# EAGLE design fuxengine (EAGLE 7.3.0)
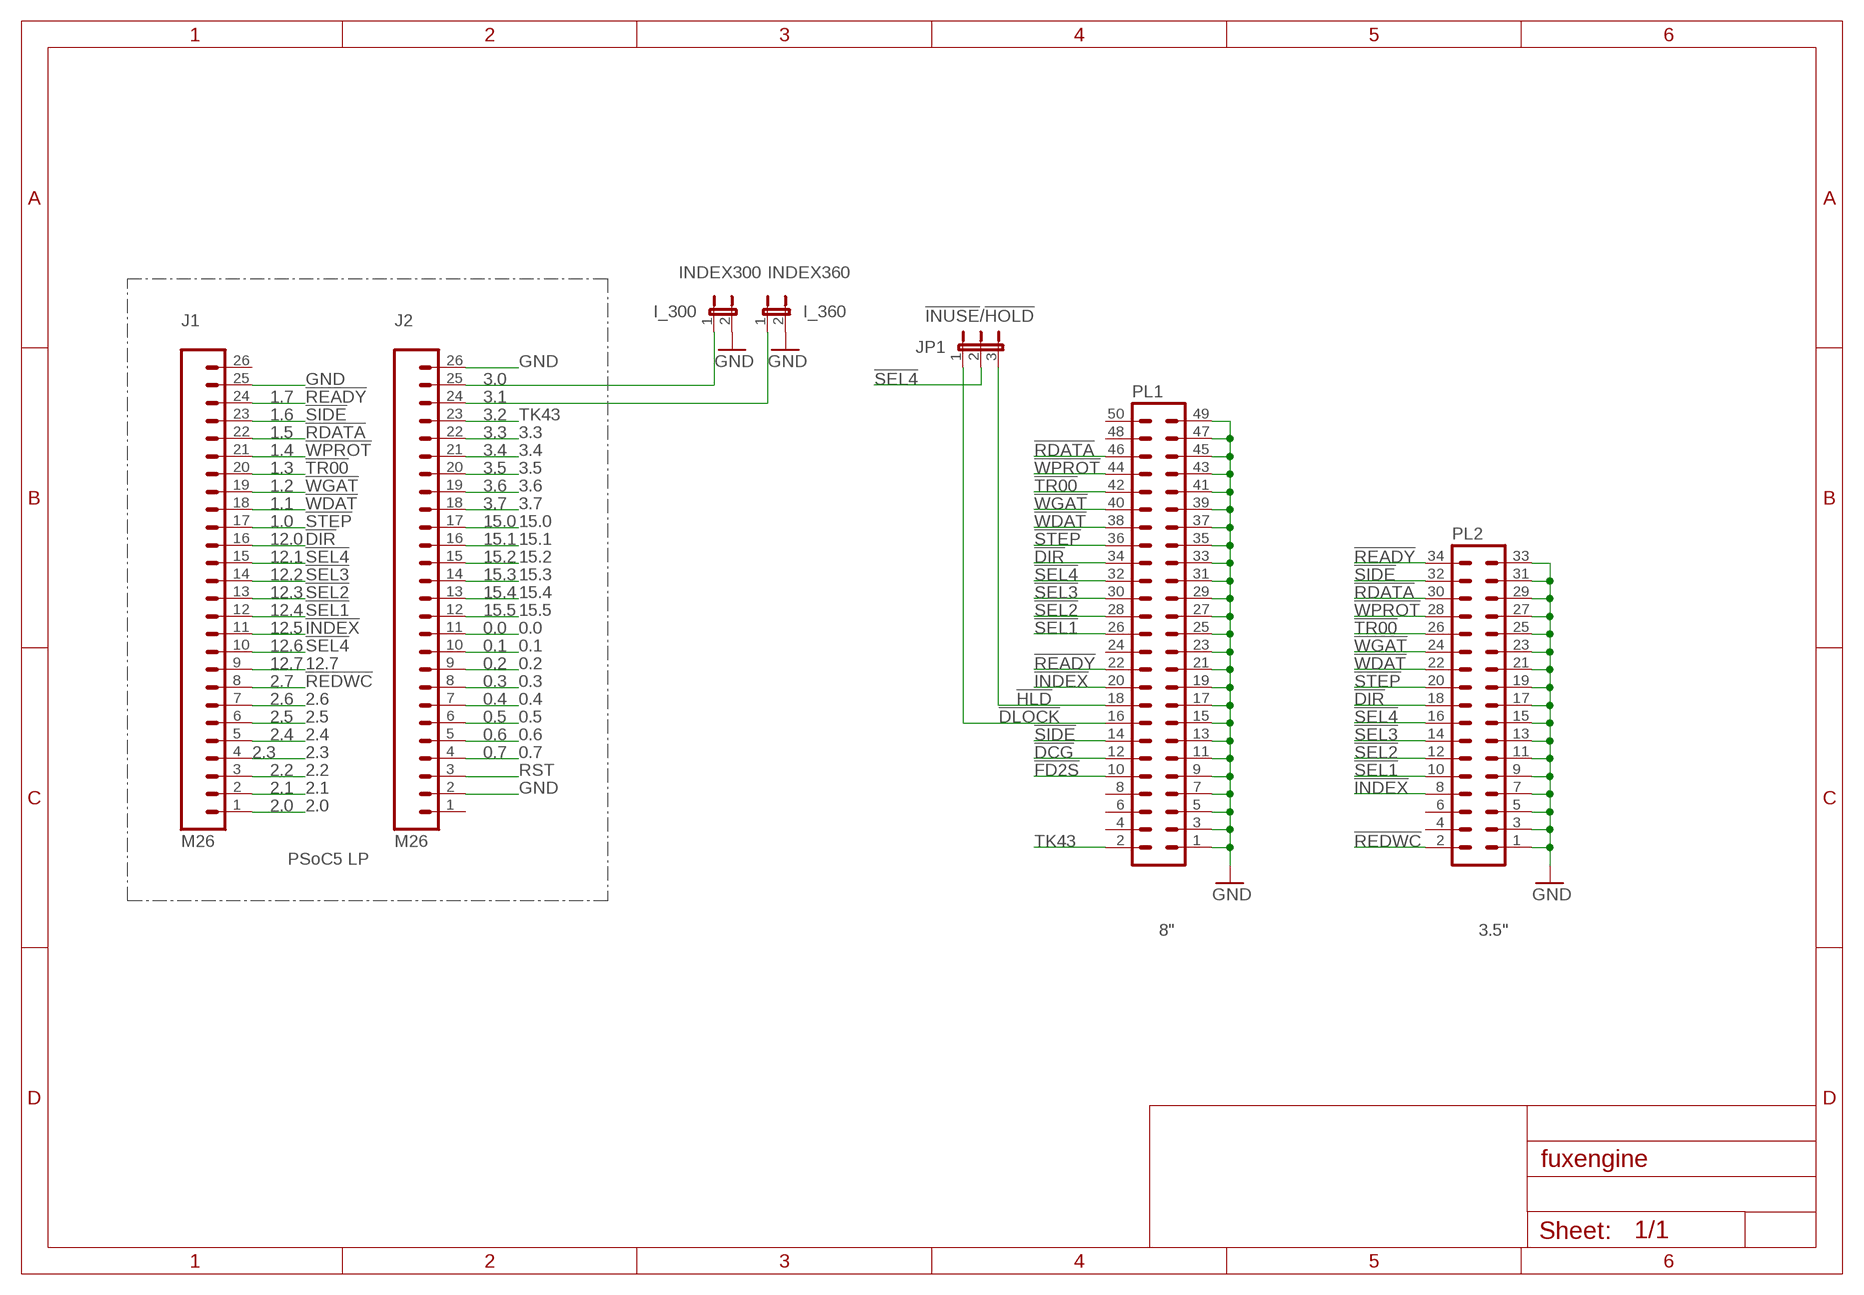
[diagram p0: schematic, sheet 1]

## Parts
I_300  JP1E  [JP1]
I_360  JP1E  [JP1]
J1  M26  [1X26]
J2  M26  [1X26]
JP1  !INUSE!/!HOLD  JP2E  [JP2]
PL1  50V  [50V]
PL2  34V  [34V]

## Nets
0.0: J2.11
0.1: J2.10
0.2: J2.9
0.3: J2.8
0.4: J2.7
0.5: J2.6
0.6: J2.5
0.7: J2.4
2.0: J1.1
2.1: J1.2
2.2: J1.3
2.3: J1.4
2.4: J1.5
2.5: J1.6
2.6: J1.7
3.3: J2.22
3.4: J2.21
3.5: J2.20
3.6: J2.19
3.7: J2.18
12.7: J1.9
15.0: J2.17
15.1: J2.16
15.2: J2.15
15.3: J2.14
15.4: J2.13
15.5: J2.12
!DCG: PL1.12
!DIR: J1.16 PL1.34 PL2.18
!DLOCK: JP1.1 PL1.16
!FD2S: PL1.10
!HLD: JP1.3 PL1.18
!INDEX: J1.11 PL1.20 PL2.8
!RDATA: J1.22 PL1.46 PL2.30
!READY: J1.24 PL1.22 PL2.34
!REDWC: J1.8 PL2.2
!SEL1: J1.12 PL1.26 PL2.10
!SEL2: J1.13 PL1.28 PL2.12
!SEL3: J1.14 PL1.30 PL2.14
!SEL4: J1.10 J1.15 JP1.2 PL1.32 PL2.16
!SIDE: J1.23 PL1.14 PL2.32
!STEP: J1.17 PL1.36 PL2.20
!TR00: J1.20 PL1.42 PL2.26
!WDAT: J1.18 PL1.38 PL2.22
!WGAT: J1.19 PL1.40 PL2.24
!WPROT: J1.21 PL1.44 PL2.28
GND: I_300.2 I_360.2 J1.25 J2.2 J2.26 PL1.1 PL1.3 PL1.5 PL1.7 PL1.9 PL1.11 PL1.13 PL1.15 PL1.17 PL1.19 PL1.21 PL1.23 PL1.25 PL1.27 PL1.29 PL1.31 PL1.33 PL1.35 PL1.37 PL1.39 PL1.41 PL1.43 PL1.45 PL1.47 PL1.49 PL2.1 PL2.3 PL2.5 PL2.7 PL2.9 PL2.11 PL2.13 PL2.15 PL2.17 PL2.19 PL2.21 PL2.23 PL2.25 PL2.27 PL2.29 PL2.31 PL2.33
INDEX300: I_300.1 J2.25
INDEX360: I_360.1 J2.24
RST: J2.3
TK43: J2.23 PL1.2
Unconnected: J1.26 J2.1 PL1.4 PL1.6 PL1.8 PL1.24 PL1.48 PL1.50 PL2.4 PL2.6

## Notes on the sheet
- 3.0
- 1.7 | 3.1
- 1.6 | 3.2
- 1.5 | 3.3
- 1.4 | 3.4
- 1.3 | 3.5
- 1.2 | 3.6
- 1.1 | 3.7
- 1.0 | 15.0
- 12.0 | 15.1
- 12.1 | 15.2
- 12.2 | 15.3
- 12.3 | 15.4
- 12.4 | 15.5
- 12.5 | 0.0
- 12.6 | 0.1
- 12.7 | 0.2
- 2.7 | 0.3
- 2.6 | 0.4
- 2.5 | 0.5
- 2.4 | 0.6
- 2.3 | 0.7
- 2.2
- 2.1
- 2.0
- PSoC5 LP
- 8" | 3.5"

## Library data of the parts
I_300 I_360 = jumper:JP1E: JUMPER
J1 J2 = SparkFun-Connectors:M26
JP1 = jumper:JP2E: JUMPER
PL1 = con-harting-v:50V: CONNECTOR; OC_FARNELL: unknown; OC_NEWARK: unknown
PL2 = con-harting-v:34V: CONNECTOR; OC_FARNELL: unknown; OC_NEWARK: unknown

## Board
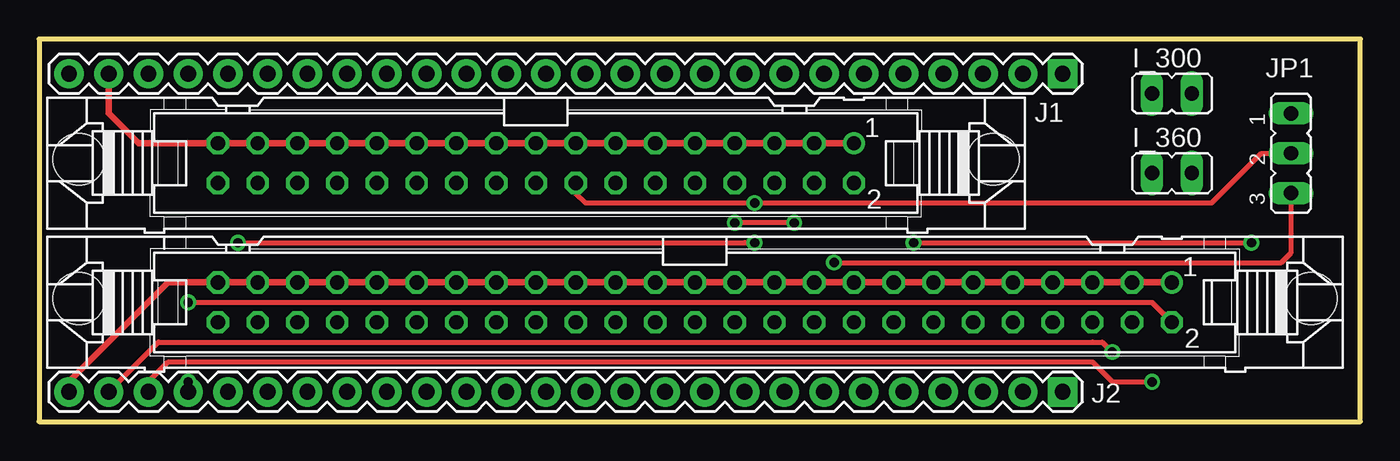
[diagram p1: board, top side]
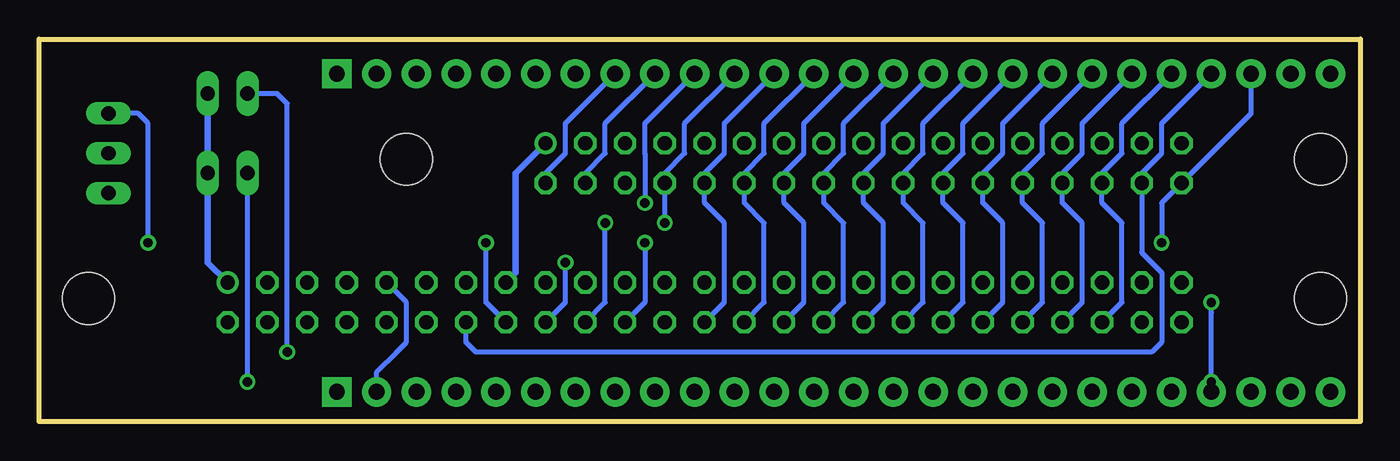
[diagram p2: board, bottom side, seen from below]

Size 84.44 x 24.43 mm. Coordinates in mm from the lower left corner, seen from the top.
Outline: 0,0 84.44,0 84.44,24.43 0,24.43 0,0
Copper layers (1*16): Top 0.035mm / dielectric 1.5mm / Bottom 0.035mm
Design rules "default": minimum track width 10mil, minimum drill 24mil, track to track 8mil, track to pad 8mil, pad to pad 8mil, via to via 8mil, smd to smd 8mil, copper to edge 40mil, drill to drill 8mil, minimum pad ring 10mil, minimum via ring 8mil, stop-mask expansion 4mil, vias tented up to drill 0mil, thermal gap 10mil

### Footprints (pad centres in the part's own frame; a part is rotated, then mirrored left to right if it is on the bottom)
JP1 = drill 0.914 long: 1 0,-1.27; 2 0,1.27
1X26 = drill 1.016 pad 1.88 square: 1 0,0 | drill 1.016 pad 1.88: 2 2.54,0; 3 5.08,0; 4 7.62,0; 5 10.16,0; 6 12.7,0; 7 15.24,0; 8 17.78,0; 9 20.32,0; 10 22.86,0; 11 25.4,0; 12 27.94,0; 13 30.48,0; 14 33.02,0; 15 35.56,0; 16 38.1,0; 17 40.64,0; 18 43.18,0; 19 45.72,0; 20 48.26,0; 21 50.8,0; 22 53.34,0; 23 55.88,0; 24 58.42,0; 25 60.96,0; 26 63.5,0
JP2 = drill 0.914 long: 1 -2.54,0; 2 0,0; 3 2.54,0
50V = drill 0.914: 1 -30.48,-1.27 | drill 0.914 octagon: 2 -30.48,1.27; 3 -27.94,-1.27; 4 -27.94,1.27; 5 -25.4,-1.27; 6 -25.4,1.27; 7 -22.86,-1.27; 8 -22.86,1.27; 9 -20.32,-1.27; 10 -20.32,1.27; 11 -17.78,-1.27; 12 -17.78,1.27; 13 -15.24,-1.27; 14 -15.24,1.27; 15 -12.7,-1.27; 16 -12.7,1.27; 17 -10.16,-1.27; 18 -10.16,1.27; 19 -7.62,-1.27; 20 -7.62,1.27; 21 -5.08,-1.27; 22 -5.08,1.27; 23 -2.54,-1.27; 24 -2.54,1.27; 25 0,-1.27; 26 0,1.27; 27 2.54,-1.27; 28 2.54,1.27; 29 5.08,-1.27; 30 5.08,1.27; 31 7.62,-1.27; 32 7.62,1.27; 33 10.16,-1.27; 34 10.16,1.27; 35 12.7,-1.27; 36 12.7,1.27; 37 15.24,-1.27; 38 15.24,1.27; 39 17.78,-1.27; 40 17.78,1.27; 41 20.32,-1.27; 42 20.32,1.27; 43 22.86,-1.27; 44 22.86,1.27; 45 25.4,-1.27; 46 25.4,1.27; 47 27.94,-1.27; 48 27.94,1.27; 49 30.48,-1.27; 50 30.48,1.27 | hole 3.302: 39.37,-0.254; -39.37,-0.254
34V = drill 0.914: 1 -20.32,-1.27 | drill 0.914 octagon: 2 -20.32,1.27; 3 -17.78,-1.27; 4 -17.78,1.27; 5 -15.24,-1.27; 6 -15.24,1.27; 7 -12.7,-1.27; 8 -12.7,1.27; 9 -10.16,-1.27; 10 -10.16,1.27; 11 -7.62,-1.27; 12 -7.62,1.27; 13 -5.08,-1.27; 14 -5.08,1.27; 15 -2.54,-1.27; 16 -2.54,1.27; 17 0,-1.27; 18 0,1.27; 19 2.54,-1.27; 20 2.54,1.27; 21 5.08,-1.27; 22 5.08,1.27; 23 7.62,-1.27; 24 7.62,1.27; 25 10.16,-1.27; 26 10.16,1.27; 27 12.7,-1.27; 28 12.7,1.27; 29 15.24,-1.27; 30 15.24,1.27; 31 17.78,-1.27; 32 17.78,1.27; 33 20.32,-1.27; 34 20.32,1.27 | hole 3.302: 29.21,-0.254; -29.21,-0.254

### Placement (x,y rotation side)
I_300  72.39,20.96 270 top
I_360  72.39,15.88 270 top
J1  65.41,22.23 180 top
J2  65.41,1.91 180 top
JP1  80.01,17.14 270 top
PL1  41.91,7.62 180 top
PL2  31.75,16.51 180 top

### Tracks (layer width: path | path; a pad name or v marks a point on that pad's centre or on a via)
12.7
  Bottom 0.305: 49.53,15.88 48.26,17.14 48.26,19.05 J1.9
!DIR
  Bottom 0.305: PL1.34 30.48,7.62 30.48,12.7 31.75,13.97 PL2.18 31.75,15.88 30.48,17.14 30.48,19.05 J1.16
!DLOCK  (via drill 0.6)
  Top 0.305: v55.88,11.43 v77.47,11.43
  Bottom 0.305: PL1.16 55.88,7.62 55.88,8.89 v55.88,11.43 | v77.47,11.43 77.47,19.05 78.1,19.68 JP1.1
!HLD  (via drill 0.6)
  Top 0.305: v50.8,10.16 79.38,10.16 80.01,10.8 JP1.3
  Bottom 0.305: PL1.18 50.8,7.62 v50.8,10.16
!INDEX  (via drill 0.6)
  Top 0.305: v48.26,12.7 v44.45,12.7
  Bottom 0.305: J1.11 43.18,19.05 43.18,17.14 44.45,15.88 PL2.8 v44.45,12.7 | PL1.20 48.26,7.62 v48.26,12.7
!RDATA
  Bottom 0.305: PL1.46 15.24,7.62 15.24,12.7 16.51,13.97 PL2.30 16.51,15.88 15.24,17.14 15.24,19.05 J1.22
!READY  (via drill 0.6)
  Top 0.305: v12.7,11.43 45.09,11.43 v45.72,11.43
  Bottom 0.305: J1.24 6.98,19.68 PL2.34 12.7,13.97 v12.7,11.43 | v45.72,11.43 45.72,7.62 PL1.22
!REDWC
  Bottom 0.305: PL2.2 52.07,15.88 50.8,17.14 50.8,19.05 J1.8
!SEL1
  Bottom 0.305: J1.12 40.64,19.05 40.64,17.14 41.91,15.88 PL2.10 41.91,13.97 40.64,12.7 40.64,7.62 PL1.26
!SEL2
  Bottom 0.305: PL1.28 38.1,7.62 38.1,12.7 39.37,13.97 PL2.12 39.37,15.88 38.1,17.14 38.1,19.05 J1.13
!SEL3
  Bottom 0.305: PL1.30 35.56,7.62 35.56,12.7 36.83,13.97 PL2.14 36.83,15.88 35.56,17.14 35.56,19.05 J1.14
!SEL4  (via drill 0.6)
  Top 0.305: PL2.16 34.29,14.61 34.92,13.97 v45.72,13.97 74.93,13.97 78.1,17.14 JP1.2
  Bottom 0.305: J1.10 45.72,19.05 45.72,17.14 v45.72,13.97 | PL1.32 33.02,7.62 33.02,12.7 34.29,13.97 PL2.16 34.29,15.88 33.02,17.14 33.02,19.05 J1.15
!SIDE
  Bottom 0.305: J1.23 12.7,19.05 12.7,17.14 13.97,15.88 PL2.32 13.97,10.8 12.7,9.53 12.7,5.08 13.34,4.45 56.51,4.45 57.15,5.08 PL1.14
!STEP
  Bottom 0.305: PL1.36 27.94,7.62 27.94,12.7 29.21,13.97 PL2.20 29.21,15.88 27.94,17.14 27.94,19.05 J1.17
!TR00
  Bottom 0.305: PL1.42 20.32,7.62 20.32,12.7 21.59,13.97 PL2.26 21.59,15.88 20.32,17.14 20.32,19.05 J1.20
!WDAT
  Bottom 0.305: PL1.38 25.4,7.62 25.4,12.7 26.67,13.97 PL2.22 26.67,15.88 25.4,17.14 25.4,19.05 J1.18
!WGAT
  Bottom 0.305: PL1.40 22.86,7.62 22.86,12.7 24.13,13.97 PL2.24 24.13,15.88 22.86,17.14 22.86,19.05 J1.19
!WPROT
  Bottom 0.305: PL1.44 17.78,7.62 17.78,12.7 19.05,13.97 PL2.28 19.05,15.88 17.78,17.14 17.78,19.05 J1.21
GND
  Top 0.406: J1.25 4.45,19.68 5.08,19.05 6.35,17.78 PL2.33 PL2.31 PL2.29 PL2.27 PL2.25 PL2.23 PL2.21 PL2.19 PL2.17 PL2.15 PL2.13 PL2.11 PL2.9 PL2.7 PL2.5 PL2.3 PL2.1 | PL1.1 PL1.3 PL1.5 PL1.7 PL1.9 PL1.11 PL1.13 PL1.15 PL1.17 PL1.19 PL1.21 PL1.23 PL1.25 PL1.27 PL1.29 PL1.31 PL1.33 PL1.35 PL1.37 PL1.39 PL1.41 PL1.43 PL1.45 PL1.47 PL1.49 8.25,8.89 1.9,2.54 J2.26
  Bottom 0.305: J2.2 62.87,3.18 61.59,4.45 60.96,5.08 60.96,7.62 PL1.9
  Bottom 0.406: PL2.1 53.98,15.88 53.98,9.53 PL1.15 | PL1.1 73.66,10.16 I_360.2 I_300.2
INDEX300  (via drill 0.6)
  Top 0.305: J2.25 7.62,5.08 67.31,5.08 67.94,5.08 v68.58,4.45
  Bottom 0.305: v68.58,4.45 68.58,20.32 69.22,20.96 I_300.1
INDEX360  (via drill 0.6)
  Top 0.305: J2.24 6.98,2.54 8.25,3.81 67.31,3.81 68.58,2.54 v71.12,2.54
  Bottom 0.305: v71.12,2.54 71.12,12.7 71.12,13.34 I_360.1
TK43  (via drill 0.6)
  Top 0.305: J2.23 v9.52,2.54 | v9.52,7.62 71.12,7.62 PL1.2
  Bottom 0.305: v9.52,2.54 9.52,6.98 v9.52,7.62

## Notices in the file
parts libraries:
SparkFun-Connectors: Licensing: CC v3.0 Share-Alike You are welcome to use this library for commercial purposes.
